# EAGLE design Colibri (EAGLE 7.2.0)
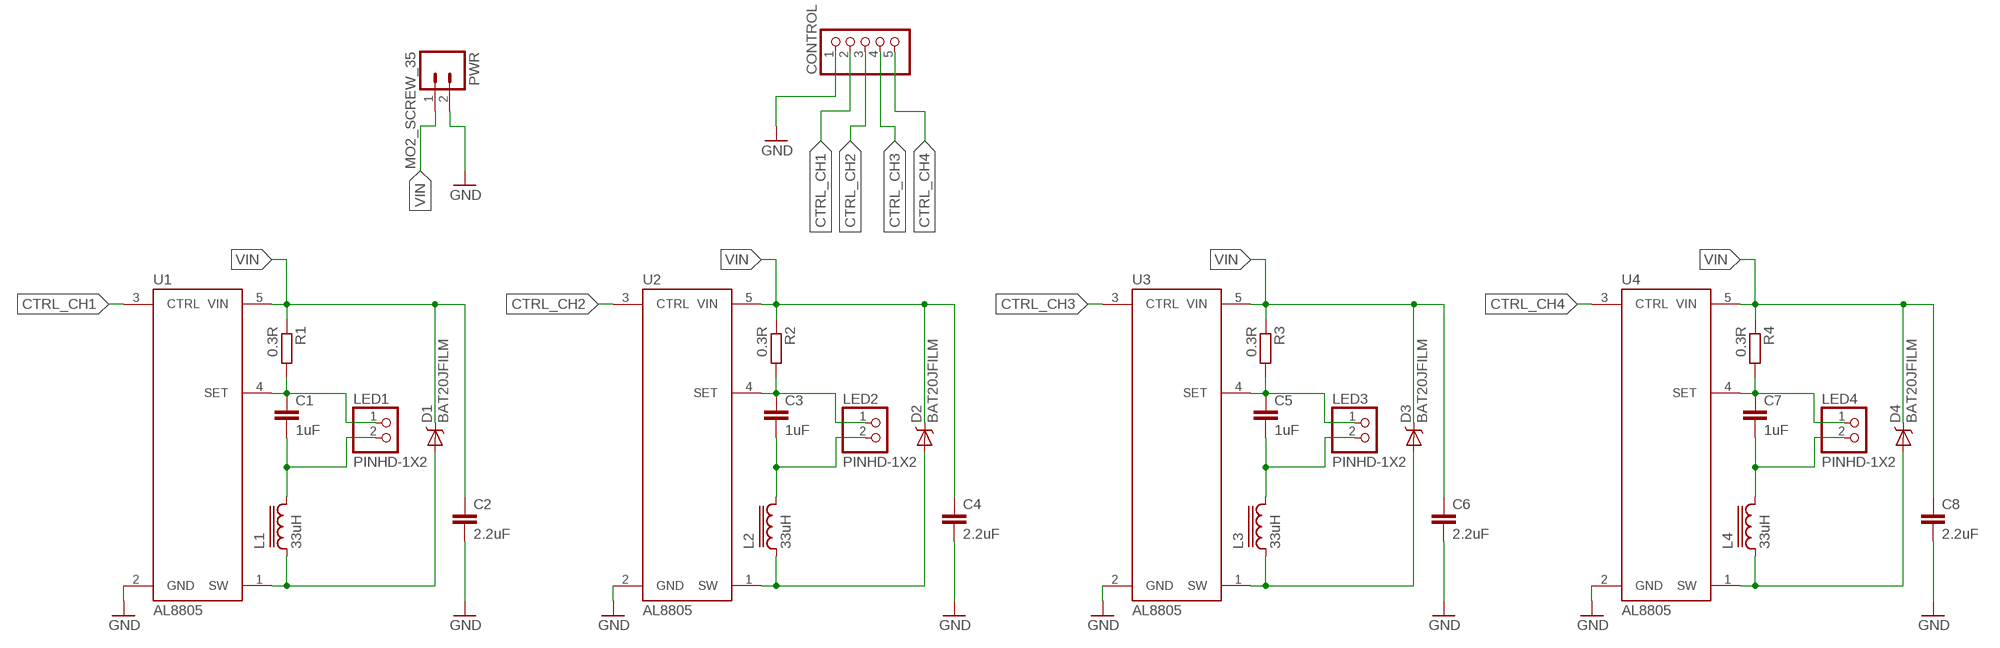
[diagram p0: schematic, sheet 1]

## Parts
C1  1uF  C0805  [C0805]
C2  2.2uF  C0805  [C0805]
C3  1uF  C0805  [C0805]
C4  2.2uF  C0805  [C0805]
C5  1uF  C0805  [C0805]
C6  2.2uF  C0805  [C0805]
C7  1uF  C0805  [C0805]
C8  2.2uF  C0805  [C0805]
CONTROL  PINHD-1X5  [1X05M]
D1  BAT20JFILM  [SOD-323]
D2  BAT20JFILM  [SOD-323]
D3  BAT20JFILM  [SOD-323]
D4  BAT20JFILM  [SOD-323]
L1  33uH  LCD75  [CD75]
L2  33uH  LCD75  [CD75]
L3  33uH  LCD75  [CD75]
L4  33uH  LCD75  [CD75]
LED1  PINHD-1X2  [1X02M]
LED2  PINHD-1X2  [1X02M]
LED3  PINHD-1X2  [1X02M]
LED4  PINHD-1X2  [1X02M]
PWR  MO2_SCREW_35  [SCREWTERMINAL-3.5MM-2-NS]
R1  0.3R  R0805  [R0805]
R2  0.3R  R0805  [R0805]
R3  0.3R  R0805  [R0805]
R4  0.3R  R0805  [R0805]
U1  AL8805  [SOT23-5]
U2  AL8805  [SOT23-5]
U3  AL8805  [SOT23-5]
U4  AL8805  [SOT23-5]

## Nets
A1: C1.1 LED1.1 R1.2 U1.4(SET)
A2: C3.1 LED2.1 R2.2 U2.4(SET)
A3: C5.1 LED3.1 R3.2 U3.4(SET)
A4: C7.1 LED4.1 R4.2 U4.4(SET)
CTRL_CH1: CONTROL.2 U1.3(CTRL)
CTRL_CH2: CONTROL.3 U2.3(CTRL)
CTRL_CH3: CONTROL.4 U3.3(CTRL)
CTRL_CH4: CONTROL.5 U4.3(CTRL)
GND: C2.2 C4.2 C6.2 C8.2 CONTROL.1 PWR.2 U1.2(GND) U2.2(GND) U3.2(GND) U4.2(GND)
IND1-1: D1.2(A) L1.P$1 U1.1(SW)
IND1-2: D2.2(A) L2.P$1 U2.1(SW)
IND1-3: D3.2(A) L3.P$1 U3.1(SW)
IND1-4: D4.2(A) L4.P$1 U4.1(SW)
K1 [power]: C1.2 L1.P$2 LED1.2
K2 [power]: C3.2 L2.P$2 LED2.2
K3 [power]: C5.2 L3.P$2 LED3.2
K4 [power]: C7.2 L4.P$2 LED4.2
VIN: C2.1 C4.1 C6.1 C8.1 D1.1(C) D2.1(C) D3.1(C) D4.1(C) PWR.1 R1.1 R2.1 R3.1 R4.1 U1.5(VIN) U2.5(VIN) U3.5(VIN) U4.5(VIN)

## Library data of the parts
C1-C8 = Max-RCL:C
CONTROL = Max-PinHead:PINHD-1X5: 5 Pin header
D1-D4 = Max-Diodes:BAT20JFILM: 23V, 1A Schottky diode, SOD-323 package; PROD_ID: DIO-11623
L1-L4 = Max-RCL:L
LED1-LED4 = Max-PinHead:PINHD-1X2
PWR = Max-Connectors:MO2_SCREW_35
R1-R4 = Max-RCL:R
U1-U4 = Max-SwitchingRegulators:AL8805

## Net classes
0 default: width 0.254 mm
1 power: width 0.508 mm

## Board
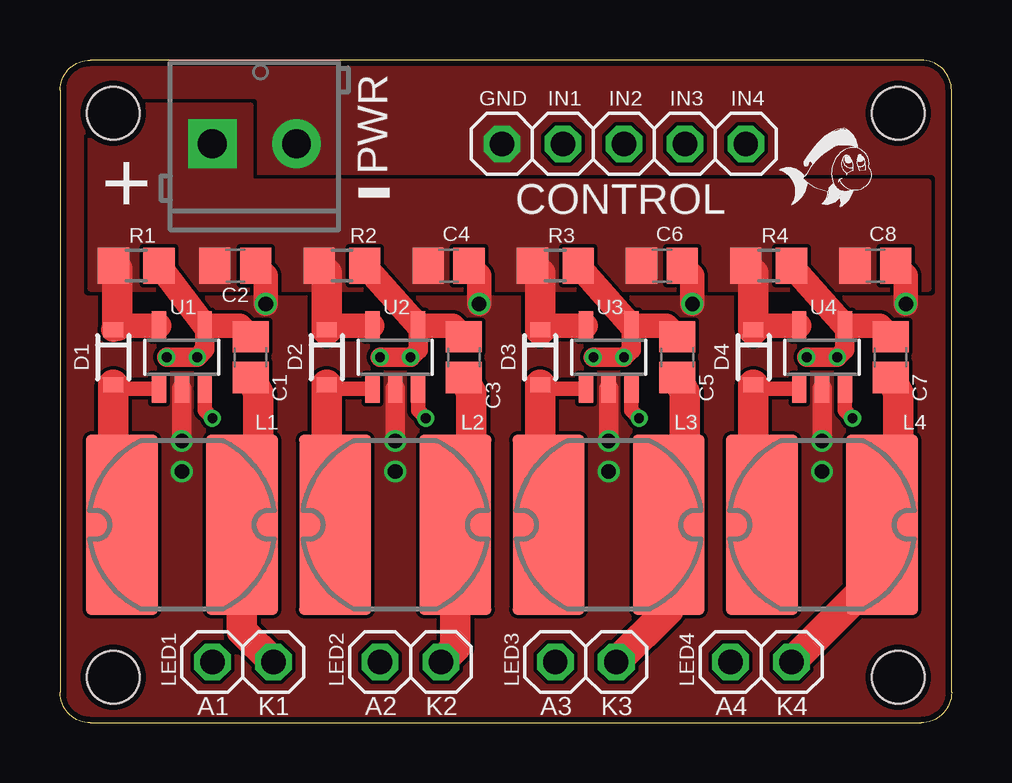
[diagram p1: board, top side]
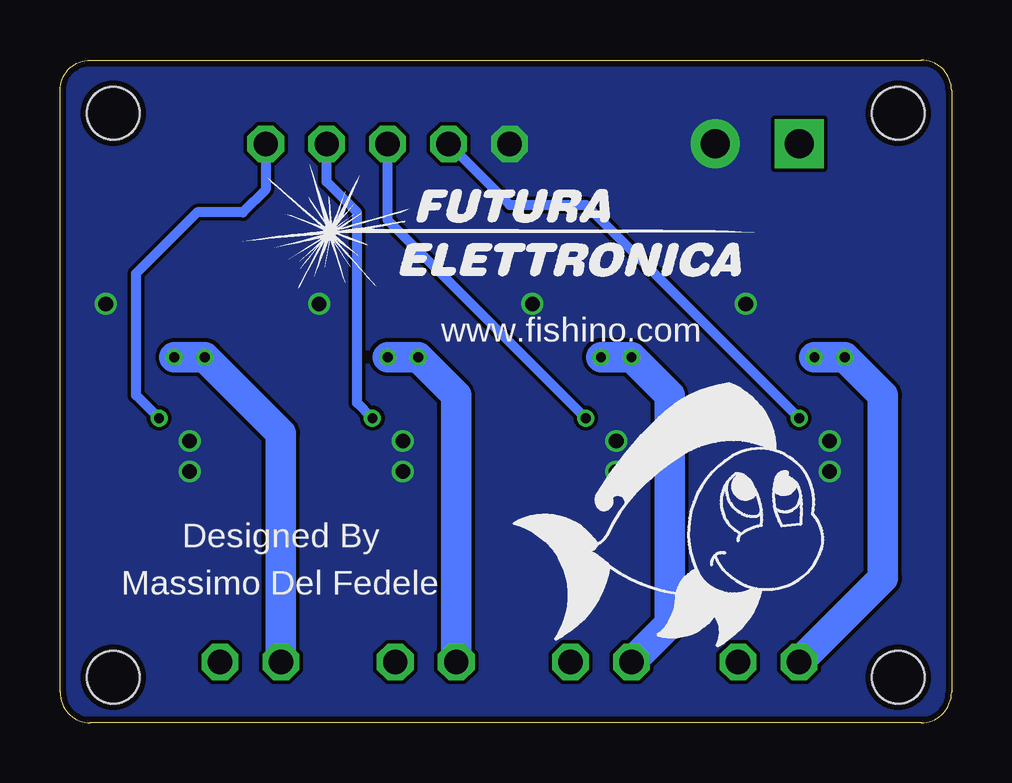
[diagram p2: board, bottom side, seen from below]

Size 37.15 x 27.62 mm. Coordinates in mm from the lower left corner, seen from the top.
Outline: 1.27,0 35.88,0 arc90 37.15,1.27 37.15,26.35 arc90 35.88,27.62 1.27,27.62 arc90 0,26.35 0,1.27 arc90 1.27,0
Copper layers (1*16): Top 0.035mm / dielectric 1.5mm / Bottom 0.035mm
Design rules "Elecrow_2-layer_eagle_rule": minimum track width 6mil, minimum drill 12mil, track to track 6mil, track to pad 6mil, pad to pad 6mil, via to via 6mil, smd to smd 0mil, copper to edge 10mil, drill to drill 10mil, minimum pad ring 10mil, minimum via ring 6mil, stop-mask expansion 2mil, vias tented up to drill 100mil, thermal gap 10mil
Holes 2.2 mm at 2.22,25.4 34.92,25.4 34.92,1.91 2.22,1.91

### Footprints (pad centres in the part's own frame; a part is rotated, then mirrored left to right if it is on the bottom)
C0805 = smd 1.3 x 1.5: 1 -0.85,0; 2 0.85,0
1X05M = drill 1.016 octagon: 1 -5.08,0; 2 -2.54,0; 3 0,0; 4 2.54,0; 5 5.08,0
SOD-323 = smd 0.63 x 0.83: 1 -1.15,0; 2 1.15,0
CD75 = smd 7.5 x 3: P$1 0,2.5; P$2 0,-2.5
1X02M = drill 1.016 octagon: 1 -1.27,0; 2 1.27,0
SCREWTERMINAL-3.5MM-2-NS = drill 1.2 pad 2.032 square: 1 0,0 | drill 1.2 pad 2.032: 2 3.5,0
R0805 = smd 1.3 x 1.5: 1 -0.95,0; 2 0.95,0
SOT23-5 = smd 0.6 x 1.2: 1 -0.95,-1.306; 2 0,-1.306; 3 0.95,-1.306; 4 0.95,1.306; 5 -0.95,1.306

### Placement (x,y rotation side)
C1  7.94,15.24 270 top
C2  7.3,19.05 0 top
C3  16.83,15.24 270 top
C4  16.19,19.05 0 top
C5  25.72,15.24 270 top
C6  25.08,19.05 0 top
C7  34.61,15.24 270 top
C8  33.97,19.05 0 top
CONTROL  23.5,24.13 0 top
D1  2.22,15.24 270 top
D2  11.11,15.24 270 top
D3  20,15.24 270 top
D4  28.89,15.24 270 top
L1  5.08,8.26 90 top
L2  13.97,8.26 90 top
L3  22.86,8.26 90 top
L4  31.75,8.26 90 top
LED1  7.62,2.54 0 top
LED2  14.61,2.54 0 top
LED3  21.91,2.54 0 top
LED4  29.21,2.54 0 top
PWR  6.35,24.13 0 top
R1  3.17,19.05 0 top
R2  11.75,19.05 0 top
R3  20.64,19.05 0 top
R4  29.53,19.05 0 top
U1  5.08,15.24 0 top
U2  13.97,15.24 0 top
U3  22.86,15.24 0 top
U4  31.75,15.24 0 top
U$1  [FISHINO]  16.51,3.49 0 bottom
U$2  [FUTURA]  29.53,18.1 0 bottom
U$3  [FISHINO_MEDIUM]  30.48,21.59 0 top

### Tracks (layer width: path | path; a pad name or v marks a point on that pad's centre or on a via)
A1  (via drill 0.41)
  Top 0.813: v4.45,15.24 v5.71,15.24 6.04,15.56 U1.4
  Top 1.016: R1.2 U1.4 7.48,16.55 C1.1
  Bottom 1.27: v5.71,15.24 v4.45,15.24 2.86,13.65 2.86,6.03 LED1.1
A2  (via drill 0.41)
  Top 0.813: v13.34,15.24 v14.61,15.24 14.92,15.55 U2.4
  Top 1.016: C3.1 16.37,16.55 U2.4 R2.2
  Bottom 1.27: v14.61,15.24 v13.34,15.24 11.75,13.65 11.75,4.13 LED2.1
A3  (via drill 0.41)
  Top 0.813: v22.23,15.24 v23.5,15.24 23.81,15.55 U3.4
  Top 1.016: C5.1 25.26,16.55 U3.4 R3.2
  Bottom 1.27: LED3.1 20.64,13.65 v22.23,15.24 v23.5,15.24
A4  (via drill 0.41)
  Top 0.813: v31.11,15.24 v32.38,15.24 32.7,15.55 U4.4
  Top 1.016: C7.1 34.15,16.55 U4.4 R4.2
  Bottom 1.27: v32.38,15.24 v31.11,15.24 27.94,12.06 LED4.1
CTRL_CH1  (via drill 0.41)
  Top 0.61: U1.3 6.03,13.02 v6.35,12.7
  Bottom 0.406: v6.35,12.7 15.24,21.59 18.41,21.59 CONTROL.2
CTRL_CH2  (via drill 0.41)
  Top 0.61: U2.3 14.92,13.02 v15.24,12.7
  Bottom 0.406: v15.24,12.7 23.5,20.95 CONTROL.3
CTRL_CH3  (via drill 0.41)
  Top 0.61: U3.3 23.81,13.02 v24.13,12.7
  Bottom 0.406: v24.13,12.7 24.77,13.34 24.77,21.27 26.04,22.54 CONTROL.4
CTRL_CH4  (via drill 0.41)
  Top 0.61: U4.3 32.7,13.02 v33.02,12.7
  Bottom 0.406: v33.02,12.7 33.97,13.65 33.97,18.73 31.43,21.27 29.53,21.27 28.57,22.23 CONTROL.5
GND  (via drill 0.61)
  Top 0.813: U1.2 v5.08,11.75 | U2.2 v13.97,11.75 | U3.2 v22.86,11.75 | U4.2 v31.75,11.75
  Top 1.016: v8.57,17.46 8.57,18.63 C2.2 | v17.46,17.46 17.46,18.63 C4.2 | v26.35,17.46 26.35,18.63 C6.2 | v35.24,17.46 35.24,18.63 C8.2
  other vias: 5.08,10.48 13.97,10.48 22.86,10.48 31.75,10.48
  pour Bottom (no thermals): 0,0 37.15,0 37.15,27.62 0,27.62
  pour Top (rank 2, no thermals): 0,0 37.15,0 37.15,27.62 0,27.62
IND1-1
  Top 0.61: U1.1 2.38,13.93 D1.2
  Top 1.27: L1.P$1 2.22,8.61 D1.2
IND1-2
  Top 0.61: U2.1 11.27,13.93 D2.2
  Top 1.27: L2.P$1 11.11,8.61 D2.2
IND1-3
  Top 0.61: U3.1 20.16,13.93 D3.2
  Top 1.27: L3.P$1 20,8.61 D3.2
IND1-4
  Top 0.61: U4.1 29.05,13.93 D4.2
  Top 1.27: L4.P$1 28.89,8.61 D4.2
K1
  Top 1.27: C1.2 8.26,13.76 8.26,9.21 7.58,8.53 L1.P$2 7.58,3.85 LED1.2
K2
  Top 1.27: C3.2 17.14,13.76 17.14,9.21 16.47,8.53 L2.P$2 16.47,3.13 LED2.2
K3
  Top 1.27: C5.2 26.04,13.76 26.04,9.21 25.36,8.53 L3.P$2 25.36,4.72 LED3.2
K4
  Top 1.27: C7.2 34.92,13.76 34.92,9.21 34.25,8.53 L4.P$2 | LED4.2 34.29,6.35 34.29,8.21
  Top 1.422: 34.29,8.21 L4.P$2
VIN
  Top 1.016: U1.5 2.38,16.55 D1.1 | U2.5 11.27,16.55 D2.1 | U3.5 20.16,16.55 D3.1 | U4.5 29.05,16.55 D4.1
  Top 1.27: 2.38,16.55 2.38,18.9 R1.1 | D2.1 11.11,18.73 R2.1 | D3.1 20,18.73 R3.1 | D4.1 28.89,18.73 R4.1
  pour Top (no thermals): 1.27,18.1 36.2,18.1 36.2,22.54 7.94,22.54 7.94,25.72 1.27,25.72

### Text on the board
tNames: GND | IN1 | IN2 | IN3 | IN4 | + | - | A1 | K1 | A2 | K2 | A3 | K3 | A4 | K4
bNames: www.fishino.com | Designed By | Massimo Del Fedele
